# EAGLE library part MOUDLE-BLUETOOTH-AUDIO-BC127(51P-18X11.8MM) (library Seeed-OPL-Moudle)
317990034
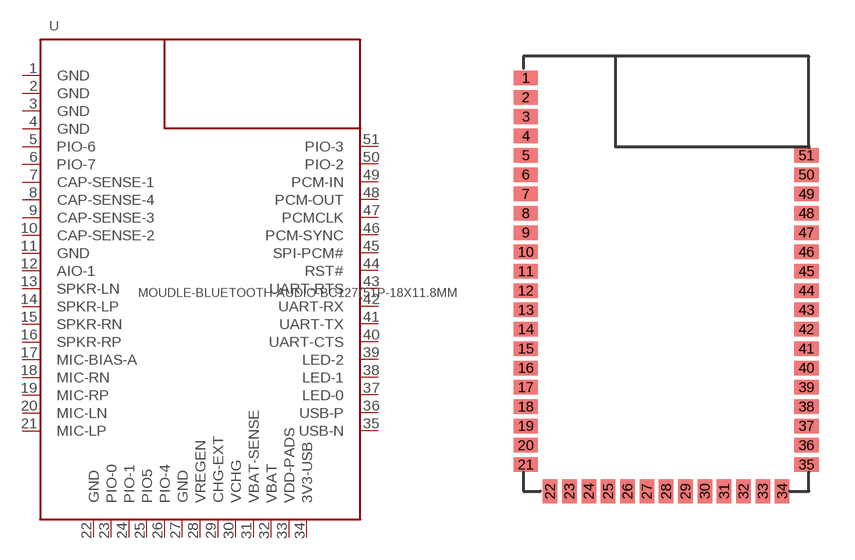
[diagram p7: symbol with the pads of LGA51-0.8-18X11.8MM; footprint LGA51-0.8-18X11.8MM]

Designator prefix U

## MOUDLE-BLUETOOTH-AUDIO-BC127(51P-18X11.8MM) (MPN: BC127; VALUE: BC127(51P 18X11.8MM))  [LGA51-0.8-18X11.8MM]
1  GND
2  GND
3  GND
4  GND
5  PIO-6
6  PIO-7
7  CAP-SENSE-1
8  CAP-SENSE-4
9  CAP-SENSE-3
10  CAP-SENSE-2
11  GND
12  AIO-1
13  SPKR-LN
14  SPKR-LP
15  SPKR-RN
16  SPKR-RP
17  MIC-BIAS-A
18  MIC-RN
19  MIC-RP
20  MIC-LN
21  MIC-LP
22  GND
23  PIO-0
24  PIO-1
25  PIO5
26  PIO-4
27  GND
28  VREGEN
29  CHG-EXT
30  VCHG
31  VBAT-SENSE
32  VBAT
33  VDD-PADS
34  3V3-USB
35  USB-N
36  USB-P
37  LED-0
38  LED-1
39  LED-2
40  UART-CTS
41  UART-TX
42  UART-RX
43  UART-RTS
44  RST#
45  SPI-PCM#
46  PCM-SYNC
47  PCMCLK
48  PCM-OUT
49  PCM-IN
50  PIO-2
51  PIO-3

## Footprint LGA51-0.8-18X11.8MM (pad centres in mm)
smd 1 x 0.6: 1 -5.8,8.1; 2 -5.8,7.3; 3 -5.8,6.5; 4 -5.8,5.7; 5 -5.8,4.9; 6 -5.8,4.1; 7 -5.8,3.3; 8 -5.8,2.5; 9 -5.8,1.7; 10 -5.8,0.9; 11 -5.8,0.1; 12 -5.8,-0.7; 13 -5.8,-1.5; 14 -5.8,-2.3; 15 -5.8,-3.1; 16 -5.8,-3.9; 17 -5.8,-4.7; 18 -5.8,-5.5; 19 -5.8,-6.3; 20 -5.8,-7.1; 21 -5.8,-7.9; 35 5.8,-7.9; 36 5.8,-7.1; 37 5.8,-6.3; 38 5.8,-5.5; 39 5.8,-4.7; 40 5.8,-3.9; 41 5.8,-3.1; 42 5.8,-2.3; 43 5.8,-1.5; 44 5.8,-0.7; 45 5.8,0.1; 46 5.8,0.9; 47 5.8,1.7; 48 5.8,2.5; 49 5.8,3.3; 50 5.8,4.1; 51 5.8,4.9
smd 0.6 x 1: 22 -4.8,-9; 23 -4,-9; 24 -3.2,-9; 25 -2.4,-9; 26 -1.6,-9; 27 -0.8,-9; 28 0,-9; 29 0.8,-9; 30 1.6,-9; 31 2.4,-9; 32 3.2,-9; 33 4,-9; 34 4.8,-9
